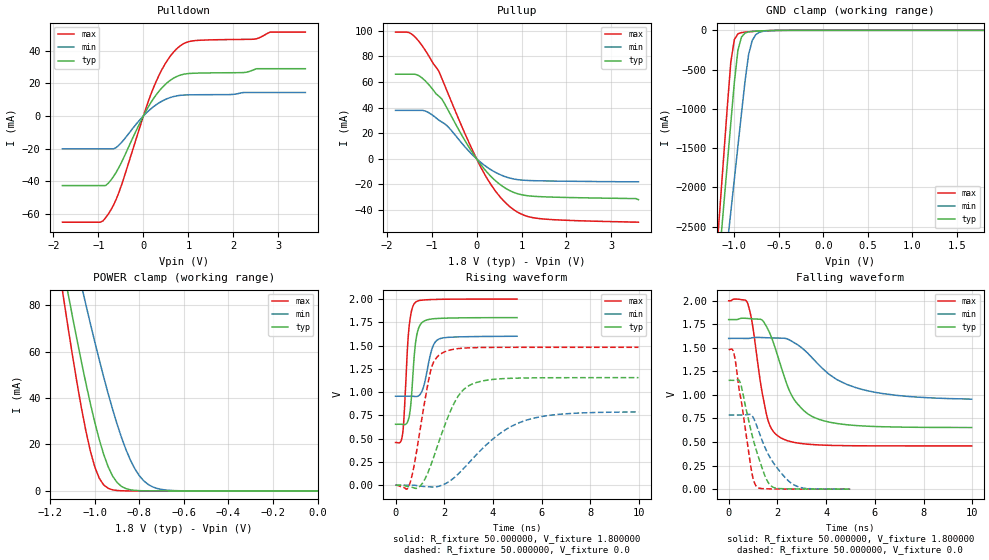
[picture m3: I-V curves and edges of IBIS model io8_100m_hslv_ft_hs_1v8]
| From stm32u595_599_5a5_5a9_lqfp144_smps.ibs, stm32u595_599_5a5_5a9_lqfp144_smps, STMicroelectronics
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|   Model io8_100m_hslv_ft_hs_1v8
[Model]  io8_100m_hslv_ft_hs_1v8
Model_type I/O
Polarity   Non-Inverting
Enable   Active-Low
Vinl =   0.540000V
Vinh =   1.260000V
Vmeas =  0.900000V
Cref =   50.000000pF
Rref =   100.000000M
Vref =   0.0V
C_comp   3.235100pF   3.233200pF   3.282800pF
[Temperature Range]   25.000000   0.140000k   -40.000000
[Pullup Reference]   1.800000V   1.600000V   2.000000V
[Pulldown Reference]   0.0V   0.0V   0.0V
[POWER Clamp Reference]   1.800000V   1.600000V   2.000000V
[GND Clamp Reference]   0.0V   0.0V   0.0V
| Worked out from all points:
|   slope of the pulldown table from 0 to 0.27 V, typ, clamps not added: 21.7 ohm
|   slope of the pullup table from 0 to 0.27 V, typ, clamps not added: 22.6 ohm
|   GND clamp passes 1 mA (typ) near -0.51 V on its own axis
|   POWER clamp passes 1 mA (typ) near -0.86 V on its own axis
|   rising waveform, R_fixture 50.000000, V_fixture 1.800000: 20-80 % time 212ps typ, 327ps min, 198ps max; typ from 0.654 V to 1.8 V
|   rising waveform, R_fixture 50.000000, V_fixture 0.0: 20-80 % time 1.02ns typ, 2.02ns min, 582ps max; typ from 0 V to 1.16 V
|   falling waveform, R_fixture 50.000000, V_fixture 1.800000: 20-80 % time 1.09ns typ, 2.02ns min, 567ps max; typ from 1.8 V to 0.654 V
|   falling waveform, R_fixture 50.000000, V_fixture 0.0: 20-80 % time 709ps typ, 988ps min, 510ps max; typ from 1.16 V to 0 V
[Pulldown]
|Voltage   I(typ)   I(min)   I(max)
-1.8V     -42.74mA   -20.21mA   -65.25mA
-960mV    -42.74mA   -20.21mA   -65.25mA
-780mV    -41.3mA    -20.21mA   -60.25mA
-540mV    -31.39mA   -17.82mA   -46.65mA
0V        -10fA      -600fA     0A
240mV     11.28mA    6.002mA    18.38mA
480mV     19.18mA    10.02mA    31.83mA
780mV     24.67mA    12.5mA     42.21mA
1.14V     26.24mA    12.99mA    46.23mA
2.46V     28.42mA    14.39mA    47.14mA
2.82V     29mA       14.39mA    51.49mA
3.6V      29mA       14.39mA    51.49mA
[Pullup]
|Voltage   I(typ)   I(min)   I(max)
-1.8V     66.02mA    37.77mA    98.95mA
-1.44V    66.02mA    37.77mA    97.32mA
-1.14V    60.87mA    37.28mA    84.78mA
-840mV    48.93mA    30.23mA    68.56mA
-660mV    39.81mA    25.95mA    53.26mA
-300mV    16.72mA    11mA       23.08mA
120mV     -5.749mA   -3.603mA   -8.316mA
420mV     -17.18mA   -10.64mA   -25.23mA
780mV     -25.61mA   -15.48mA   -38.6mA
1.08V     -28.66mA   -16.9mA    -44.47mA
1.38V     -29.58mA   -17.26mA   -46.72mA
3.6V      -32mA      -18mA      -49.6mA
[GND_clamp]
|Voltage   I(typ)   I(min)   I(max)
-1.8V     -9.707A    -9.942A    -9.774A
-1.2V     -3.309A    -4.006A    -2.864A
-1.16V    -2.777A    -3.584A    -2.239A
-1.12V    -2.246A    -3.162A    -1.614A
-1.04V    -1.186A    -2.319A    -408.6mA
-1V       -663.9mA   -1.898A    -117.8mA
-960mV    -254mA     -1.478A    -45.14mA
-920mV    -86.03mA   -1.06A     -28.58mA
-840mV    -19.12mA   -308.9mA   -18.74mA
-800mV    -13.39mA   -130.8mA   -15.31mA
-720mV    -7.948mA   -25.37mA   -9.381mA
1.8V      0A         14.95nA    0A
[POWER_clamp]
|Voltage   I(typ)   I(min)   I(max)
-1.8V     470.8mA    433.7mA    554.6mA
-1.14V    95.25mA    122.7mA    82.82mA
-1.12V    84.97mA    114mA      70.27mA
-1.06V    55.51mA    88.42mA    35.67mA
-1.04V    46.34mA    80.15mA    25.76mA
-1V       29.51mA    64.13mA    10.3mA
-940mV    10.39mA    41.86mA    1.109mA
-900mV    3.624mA    28.77mA    182.8uA
-840mV    490.7uA    13.24mA    11.35uA
-800mV    116.8uA    6.532mA    1.77uA
-740mV    13.2uA     1.723mA    109.2nA
0V        0A         18.72nA    0A
[Ramp]
| variable   typ   min   max
dV/dt_r  0.69294/1.02348n   0.47036/2.01973n   0.88872/0.58144n
dV/dt_f  0.68719/1.08427n   0.37934/1.99491n   0.92479/0.56674n
R_load = 50.000000
[Rising Waveform]
R_fixture= 50.000000
V_fixture= 1.800000
V_fixture_min= 1.600000
V_fixture_max= 2.000000
|time   V(typ)   V(min)   V(max)
0s        654.2mV    955.5mV    458.9mV
290.3ps   653.2mV    955.6mV    550.1mV
350.4ps   651.2mV    955.8mV    747.2mV
530.5ps   707.7mV    956mV      1.629V
630.6ps   879.7mV    955.9mV    1.84V
790.8ps   1.458V     953.3mV    1.957V
1.041ns   1.735V     987.6mV    1.987V
1.491ns   1.786V     1.461V     1.994V
1.742ns   1.791V     1.564V     1.996V
4.985ns   1.8V       1.6V       1.999V
[Rising Waveform]
R_fixture= 50.000000
V_fixture= 0.0
V_fixture_min= 0.0
V_fixture_max= 0.0
|time   V(typ)   V(min)   V(max)
0s        -117.6uV   -28.12uV   -97.63uV
580.6ps   -17.99mV   -33.29uV   13.45mV
1.021ns   -5.888mV   -9.782mV   619mV
1.441ns   210.7mV    -18.63mV   1.229V
1.922ns   572.5mV    1.651mV    1.421V
2.583ns   961.1mV    122.9mV    1.467V
3.323ns   1.104V     328.6mV    1.478V
4.545ns   1.146V     600.9mV    1.481V
5.646ns   1.153V     718.8mV    1.481V
9.97ns    1.155V     786.9mV    1.481V
[Falling Waveform]
R_fixture= 50.000000
V_fixture= 1.800000
V_fixture_min= 1.600000
V_fixture_max= 2.000000
|time   V(typ)   V(min)   V(max)
0s        1.8V       1.6V       1.999V
760.8ps   1.812V     1.599V     1.984V
940.9ps   1.808V     1.605V     1.802V
1.321ns   1.802V     1.609V     1.105V
1.562ns   1.721V     1.607V     783.3mV
2.102ns   1.339V     1.603V     550.2mV
2.703ns   944.5mV    1.552V     495.6mV
3.724ns   739.7mV    1.313V     468.9mV
5.746ns   667.7mV    1.042V     459.9mV
9.97ns    654.2mV    955.5mV    458.9mV
[Falling Waveform]
R_fixture= 50.000000
V_fixture= 0.0
V_fixture_min= 0.0
V_fixture_max= 0.0
|time   V(typ)   V(min)   V(max)
0s        1.155V     786.9mV    1.481V
220.2ps   1.155V     786.9mV    1.434V
460.5ps   1.139V     787mV      1.012V
951ps     583.3mV    781.2mV    175.1mV
1.151ns   398.1mV    672.9mV    25.75mV
1.491ns   139.3mV    442.1mV    4.346mV
1.692ns   47.1mV     339.1mV    3.021mV
2.573ns   2.624mV    62.61mV    873.1uV
3.073ns   1.358mV    10.5mV     433.9uV
4.985ns   -117.6uV   -28.12uV   -97.63uV
